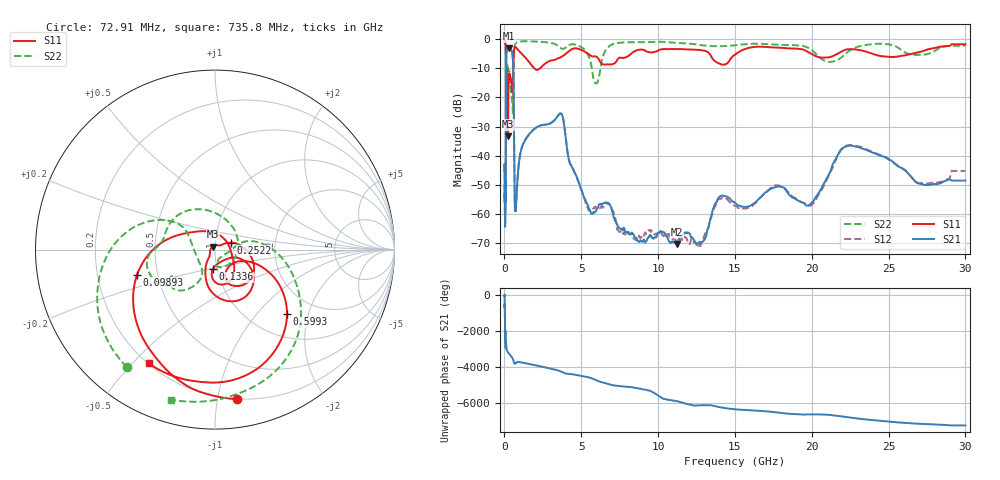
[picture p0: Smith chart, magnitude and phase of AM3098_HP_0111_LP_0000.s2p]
! Date/Time: Thu, Feb 28, 2019 8:38 AM
! Network Analyzer: Agilent Technologies E8364B Rev: A.07.50.67
! Sweep from 0.010 to 30.000 GHz, 1601 Points, Sweep Type: LOG
! Power Supply: 5.023 V, 0.002 A
# Hz S DB R 50
!freq MagS11 AngS11 MagS21 AngS21 MagS12 AngS12 MagS22 AngS22
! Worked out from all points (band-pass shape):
!   1601 points, 10 MHz to 30 GHz, reference 50 ohm
!   highest |S21| = -2.99 dB at 266.5 MHz (marker M1); lowest = -70.5 dB at 11.25 GHz (marker M2)
!   |S21| within 3 dB of the highest: 121 MHz to 534.4 MHz (413.4 MHz wide, 126 % of centre)
!   lowest |S11| = -33.4 dB at 232.8 MHz (marker M3), VSWR 1.04, Z = 48.6 + j1.61 ohm
!   |S11| at or under -10 dB: 102.2 MHz to 562.4 MHz (460.2 MHz wide, 138 % of centre); 1.955 GHz to 2.281 GHz (326.4 MHz wide, 15.4 % of centre)
!   |S22| runs from -25.5 to -0.5 dB; largest |S21 - S12| = 0.011
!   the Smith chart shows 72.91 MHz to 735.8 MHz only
!   S11 on the Smith chart (normalised r, x): 72.91 MHz: 0.20, -1.14; 98.93 MHz: 0.38, -0.13; 133.6 MHz: 0.95, -0.21; 252.2 MHz: 1.19, +0.09; 599.3 MHz: 1.45, -1.48; 735.8 MHz: 0.20, -0.56
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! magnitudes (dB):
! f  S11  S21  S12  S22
! 10 MHz  -0.3  -45.3  -43.6  -0.5
! 38.04 MHz  -0.4  -60.6  -59.5  -0.7
! 72.91 MHz  -1.5  -53.1  -52.2  -1.7
! 85.57 MHz  -2.6  -55.7  -52.2  -2.8
! 98.93 MHz  -6.8  -26.2  -26.1  -7.9
! 133.6 MHz  -19.1  -4.7  -4.6  -10.7
! 144.7 MHz  -20.4  -4.0  -4.0  -11.3
! 186.8 MHz  -11.0  -3.6  -3.5  -8.2
! 232.8 MHz  -33.4  -3.1  -3.1  -10.1
! 252.2 MHz  -20.4  -3.0  -3.0  -10.5
! 266.5 MHz  -16.3  -3.0  -3.0  -10.7
! 550.5 MHz  -12.0  -7.2  -7.2  -25.2
! 599.3 MHz  -5.4  -18.4  -18.4  -10.0
! 669.1 MHz  -2.6  -56.0  -56.2  -2.2
! 735.8 MHz  -2.7  -58.0  -57.1  -1.2
! 2.084 GHz  -10.5  -30.3  -30.2  -0.7
! 3.686 GHz  -6.0  -25.5  -25.5  -3.1
! 7.926 GHz  -6.1  -66.4  -66.7  -1.0
! 11.25 GHz  -3.3  -70.5  -69.2  -1.2
! 19.9 GHz  -4.7  -56.9  -57.3  -3.3
! 22.67 GHz  -3.4  -36.7  -36.4  -3.2
! 30 GHz  -1.7  -48.7  -45.3  -2.2
